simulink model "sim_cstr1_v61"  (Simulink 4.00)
settings: Solver=ode45  StartTime=0.0  StopTime=50  RelTol=1e-3

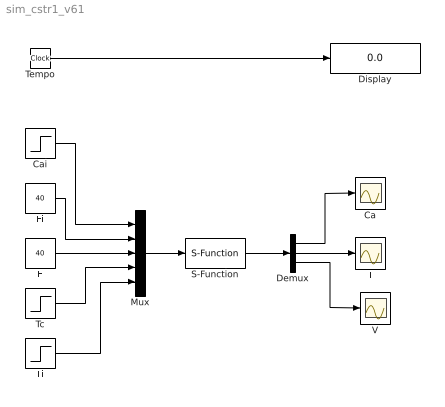
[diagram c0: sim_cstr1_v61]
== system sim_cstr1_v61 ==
  Ca : Scope
  Cai : Step  Time=0  Before=0.2  After=0.2  SampleTime=-1
  Demux : Demux  Outputs=3  BusSelectionMode=off
  Display : Display
  F : Constant  Value=40
  Fi : Constant  Value=40
  Mux : Mux  Inputs=5
  S-Function : S-Function  FunctionName=reator  Parameters=U A DeltaH ro Cp E R k0  PortCounts=[]  SFunctionModules=''  mask{k0=7.08e10, R=1.99, E=30000, Cp=0.75, ro=50, DeltaH=-30000, A=250, U=150}
      mask prompts: E "Energia de Ativação:"; ro "Densidade:"; DeltaH "Calor de Reação:"; A "Área de Troca Térmica:"
      mask help: Reator CSTR
  T : Scope
  Tc : Step  Time=0  Before=580  After=580  SampleTime=-1
  Tempo : Clock
  Ti : Step  Time=0  Before=560  After=560  SampleTime=-1
  V : Scope
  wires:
  Cai/1 -> Mux/1
  Fi/1 -> Mux/2
  F/1 -> Mux/3
  Tc/1 -> Mux/4
  Ti/1 -> Mux/5
  Mux/1 -> S-Function/1
  S-Function/1 -> Demux/1
  Demux/1 -> Ca/1
  Demux/2 -> T/1
  Demux/3 -> V/1
  Tempo/1 -> Display/1
